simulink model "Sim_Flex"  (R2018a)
settings: Solver=ode3  StartTime=0.0  StopTime=30000  FixedStep=Ts  RelTol=1e-3  EnableMultiTasking=on
InitFcn:
  | run
StopFcn:
  | pl
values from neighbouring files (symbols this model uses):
  atto = [0, 0, -0]'*d2r    [run.m]
  ini = [wb0; atto; Hco]    [run.m]
  Kq1 = I22*ww^2 - 3*wo2*(I11-I33)    [run.m]
  Kq2 = 2*I22*zet*ww    [run.m]
  Kqi = 0.0005    [run.m]
  Kr1 = (0.1*I11*I33*zet^2/Hy0) - sqrt( ((0.01^zet^4*I11^2*I33^2)/Hy0^2)+(4*I11*I33*zet^2) )    [run.m]
  Kr2 = 0.05*Kr1    [run.m]
  Kr3 = 0.04*zet*(Kr2-Hy0) * sqrt(abs(Hy0/(I11*I33)))    [run.m]
  r2d = 180/pi    (= 57.2957795131)    [pl.m]    (also in run.m; plf.m; runf.m; pl2.m)
  Tbs = (wo2)*[-2*I32, 3*I31, -I12]'    [run.m]
  Ts = 0.001    [run.m]    (also in runf.m = 0.0005)
  wb0 = [0.0, -wo, 0.0]'    [run.m]
undefined symbols (not defined in the file or in its folder): Avf, Bvf, Cvf, den, DiscIntNeverNeededParam, Dvf, num, Spacecraft, Wheel_Dynamics
libraries: simulink x3

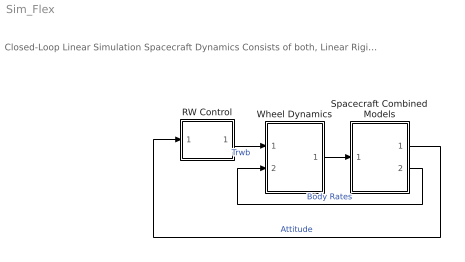
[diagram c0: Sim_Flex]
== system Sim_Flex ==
  note: Closed-Loop Linear Simulation Spacecraft Dynamics Consists of both, Linear Rigid plus Flex Subsystems
  RW Control : Subsystem
  Spacecraft Combined Models : Subsystem
  Wheel Dynamics : Subsystem
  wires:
  RW Control/1(Tc) -> Wheel Dynamics/1(Twi)  "Trwb"
  Wheel Dynamics/1(Tcb) -> Spacecraft Combined Models/1(Trw)
  Spacecraft Combined Models/2(wb) -> Wheel Dynamics/2(wb)  "Body Rates"
  Spacecraft Combined Models/1(attit) -> RW Control/1(atti)  "Attitude"

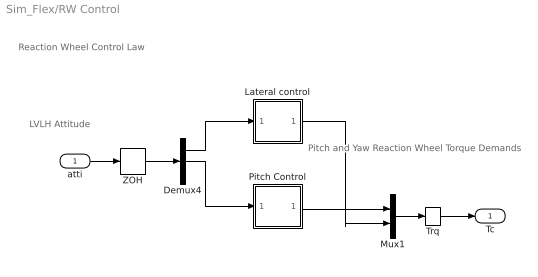
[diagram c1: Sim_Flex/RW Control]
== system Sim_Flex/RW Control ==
  note: Pitch and Yaw Reaction Wheel Torque Demands
  note: LVLH Attitude
  note: Reaction Wheel Control Law
  atti : Inport
  Demux4 : Demux  Outputs=3
  Lateral control : Subsystem
  Mux1 : Mux  Inputs=2
  Pitch Control : Subsystem
  Trq : Memory
  ZOH : ZeroOrderHold  SampleTime=Ts
  Tc : Outport
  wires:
  Demux4/1 -> Lateral control/1(phi)
  Pitch Control/1(Tcy) -> Mux1/1
  Demux4/2 -> Pitch Control/1(the)
  Lateral control/1(Tcz) -> Mux1/2
  atti/1 -> ZOH/1
  Mux1/1 -> Trq/1
  ZOH/1 -> Demux4/1
  Trq/1 -> Tc/1

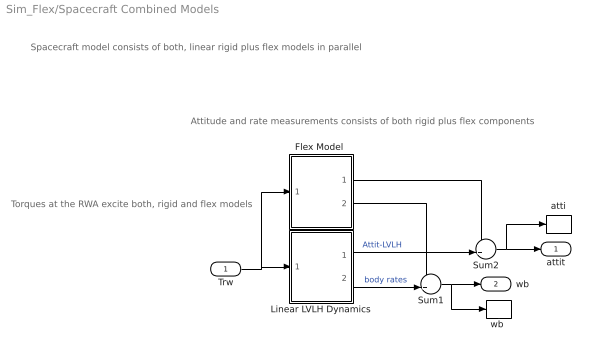
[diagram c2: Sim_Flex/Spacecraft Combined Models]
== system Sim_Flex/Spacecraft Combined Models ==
  note: Torques at the RWA excite both, rigid and flex models
  note: Spacecraft model consists of both, linear rigid plus flex models in parallel
  note: Attitude and rate measurements consists of both rigid plus flex components
  Trw : Inport
  "Flex Model " : Subsystem
  Linear LVLH Dynamics : Subsystem
  Sum1 : Sum  Inputs=++|
  Sum2 : Sum  Inputs=++|
  atti : ToWorkspace  VariableName=atti  SampleTime=-1
  "wb " : ToWorkspace  VariableName=wb  SampleTime=-1
  attit : Outport
  wb : Outport  Port=2
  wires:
  "Flex Model "/2(wb-flx) -> Sum1/1
  Linear LVLH Dynamics/2(wb) -> Sum1/2  "body rates"
  Sum1/1 -> wb/1, "wb "/1
  Sum2/1 -> attit/1, atti/1
  Linear LVLH Dynamics/1(atti-lv) -> Sum2/2  "Attit-LVLH"
  "Flex Model "/1(att-flx) -> Sum2/1
  Trw/1 -> Linear LVLH Dynamics/1(Tsc), "Flex Model "/1(Trwi)

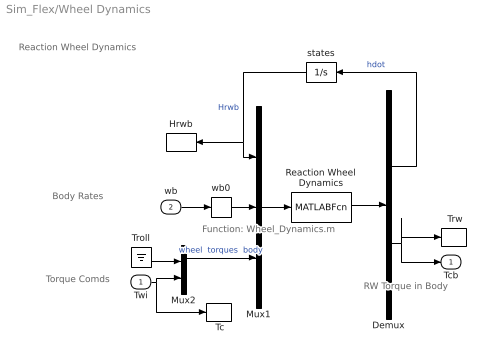
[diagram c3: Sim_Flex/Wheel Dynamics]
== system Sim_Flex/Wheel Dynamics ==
  note: Torque Comds
  note: RW Torque in Body
  note: Body Rates
  note: Reaction Wheel Dynamics
  note: Function: Wheel_Dynamics.m
  Twi : Inport
  wb : Inport  Port=2
  " Tc" : ToWorkspace  VariableName=Tc  SampleTime=-1
  " Trw" : ToWorkspace  VariableName=Trw  SampleTime=-1
  Demux : Demux  Outputs=[3, 3]
  Hrwb : ToWorkspace  VariableName=Hrwb  SampleTime=-1
  Mux1 : Mux  Inputs=[3, 3, 3]
  Mux2 : Mux  Inputs=[1,2]
  Reaction Wheel Dynamics : MATLABFcn  MATLABFcn=Wheel_Dynamics( u(1:3), u(4:6), u(7:9) )  OutputDimensions=3+3
  Troll : Ground
  states : Integrator
  wb0 : Memory  InitialCondition=wb0
  Tcb : Outport
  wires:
  wb0/1 -> Mux1/2
  Troll/1 -> Mux2/1
  Twi/1 -> Mux2/2, " Tc"/1
  Mux1/1 -> Reaction Wheel Dynamics/1
  Reaction Wheel Dynamics/1 -> Demux/1
  Demux/2 -> Tcb/1, " Trw"/1
  Mux2/1 -> Mux1/3  "wheel  torques  body"
  wb/1 -> wb0/1
  Demux/1 -> states/1  "hdot"
  states/1 -> Hrwb/1, Mux1/1  "Hrwb"

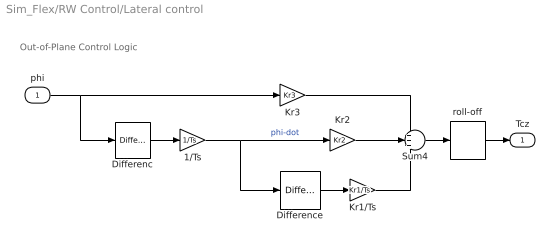
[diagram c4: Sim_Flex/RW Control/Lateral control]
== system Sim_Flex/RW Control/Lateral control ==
  note: Out-of-Plane Control Logic
  phi : Inport
  1/Ts : Gain  Gain=1/Ts
  Differenc : simulink/Discrete/Difference  ICPrevInput=atto(1)  InputProcessing=Inherited  OutMin=[]  OutMax=[]  OutDataType=sfix(16)  OutScaling=2^-10  DoSatur=off
  Difference : simulink/Discrete/Difference  ICPrevInput=0.0  InputProcessing=Inherited  OutMin=[]  OutMax=[]  OutDataType=sfix(16)  OutScaling=2^-10  DoSatur=off
  Kr1/Ts : Gain  Gain=Kr1/Ts
  Kr2 : Gain  Gain=Kr2
  Kr3 : Gain  Gain=Kr3
  Sum4 : Sum  Inputs=+++
  roll-off : DiscreteTransferFcn  Numerator=[num]  Denominator=[den]  SampleTime=Ts
  Tcz : Outport
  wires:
  Kr3/1 -> Sum4/1
  Kr2/1 -> Sum4/2
  Kr1/Ts/1 -> Sum4/3
  phi/1 -> Kr3/1, Differenc/1
  Sum4/1 -> roll-off/1
  Difference/1 -> Kr1/Ts/1
  Differenc/1 -> 1/Ts/1
  1/Ts/1 -> Kr2/1, Difference/1  "phi-dot"
  roll-off/1 -> Tcz/1

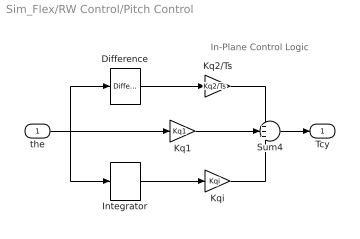
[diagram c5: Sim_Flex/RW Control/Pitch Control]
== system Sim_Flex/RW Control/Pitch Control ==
  note: In-Plane Control Logic
  the : Inport
  Difference : simulink/Discrete/Difference  ICPrevInput=atto(2)  InputProcessing=Inherited  OutMin=[]  OutMax=[]  OutDataType=sfix(16)  OutScaling=2^-10  DoSatur=off
  Integrator : DiscreteIntegrator  InitialCondition=atto(2)  SampleTime=Ts  ICPrevOutput=DiscIntNeverNeededParam  ICPrevScaledInput=DiscIntNeverNeededParam
  Kq1 : Gain  Gain=Kq1
  Kq2/Ts : Gain  Gain=Kq2/Ts
  Kqi : Gain  Gain=Kqi
  Sum4 : Sum  Inputs=+++
  Tcy : Outport
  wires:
  Kq1/1 -> Sum4/2
  Sum4/1 -> Tcy/1
  Kq2/Ts/1 -> Sum4/1
  the/1 -> Kq1/1, Integrator/1, Difference/1
  Kqi/1 -> Sum4/3
  Integrator/1 -> Kqi/1
  Difference/1 -> Kq2/Ts/1

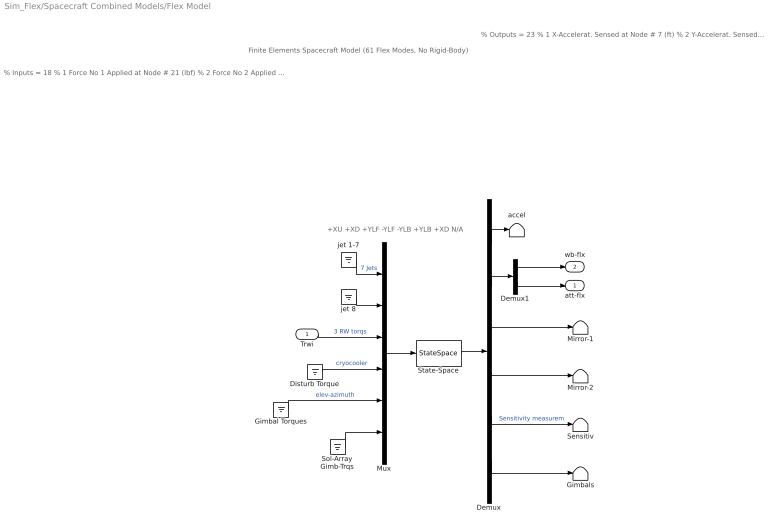
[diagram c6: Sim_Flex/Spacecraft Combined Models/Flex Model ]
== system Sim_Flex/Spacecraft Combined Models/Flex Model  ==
  note: +XU +XD +YLF -YLF -YLB +YLB +XD N/A
  note: % Outputs = 23 % 1 X-Accelerat. Sensed at Node # 7 (ft) % 2 Y-Accelerat. Sensed at Node # 7 (ft) % 3 X-Rot. Rate Sensed at Node # 6 (radian) % 4 Y-Rot. Rate Sensed at Node # 6 (radian) % 5 Z-Rot. Rate Sensed at Node # 6 (radian) % 6 X-Rotation Sensed at Node # 6 (radian) % 7 Y-Rotation Sensed at Node # 6 (radian) % 8 Z-Rotation Sensed at Node # 6 (radian) % 9 Y-Rotation Sensed at Node # 9 (radian) % 10 Z-Rotation Sensed at Node # 9 (radian) % 11 Y-Rotation Sensed at Node # 10 (radian) % 12 Z-Rotation Sensed at Node # 10 (radian) % 13 X-Rotation Sensed at Node # 11 (radian) % 14 Y-Rotation Sensed at Node # 12 (radian) % 15 Z-Rotation Sensed at Node # 13 (radian) % 16 Rotation Angle at Gimbal No 1 in (radians) % 17 Rotation Rate at Gimbal No 1 in (rad/sec) % 18 Rotation Angle at Gimbal No 2 in (radians) % 19 Rotation Rate at Gimbal No 2 in (rad/sec) % 20 Rotation Angle at Gimbal No 3 in (radians) % 21 Rotation Rate at Gimbal No 3 in (rad/sec) % 22 Rotation Angle at Gimbal No 4 in (radians) % 23 Rotation Rate at Gimbal No 4 in (rad/sec)
  note: % Inputs = 18 % 1 Force No 1 Applied at Node # 21 (lbf) % 2 Force No 2 Applied at Node # 22 (lbf) % 3 Force No 3 Applied at Node # 23 (lbf) % 4 Force No 4 Applied at Node # 24 (lbf) % 5 Force No 5 Applied at Node # 25 (lbf) % 6 Force No 6 Applied at Node # 26 (lbf) % 7 Force No 7 Applied at Node # 27 (lbf) % 8 Force No 8 Applied at Node # 28 (lbf) % 9 Torque No 1 Applied at Node # 17 (ft-lb) % 10 Torque No 2 Applied at Node # 18 (ft-lb) % 11 Torque No 3 Applied at Node # 19 (ft-lb) % 12 Torque No 4 Applied at Node # 8 (ft-lb) % 13 Torque No 5 Applied at Node # 8 (ft-lb) % 14 Torque No 6 Applied at Node # 8 (ft-lb) % 15 Control Torque at Gimbal No 1 in (ft-lb) % 16 Control Torque at Gimbal No 2 in (ft-lb) % 17 Control Torque at Gimbal No 3 in (ft-lb) % 18 Control Torque at Gimbal No 4 in (ft-lb)
  note: Finite Elements Spacecraft Model (61 Flex Modes, No Rigid-Body)
  Trwi : Inport
  Demux : Demux  Outputs="[2, 6, 2,2,3,  8]"
  Demux1 : Demux  Outputs=[3, 3]
  Disturb Torque : Ground
  Gimbal Torques : Ground
  Gimbals : Terminator
  Mirror-1 : Terminator
  Mirror-2 : Terminator
  Mux : Mux  Inputs=[7,1,3,3,2,2]
  Sensitiv : Terminator
  Sol-Array Gimb-Trqs : Ground
  State-Space : StateSpace  A=Avf  B=Bvf  C=Cvf  D=Dvf  InitialCondition=0
  accel : Terminator
  jet 1-7 : Ground
  jet 8 : Ground
  att-flx : Outport
  wb-flx : Outport  Port=2
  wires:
  Demux1/2 -> att-flx/1
  Demux/4 -> Mirror-2/1
  Demux/3 -> Mirror-1/1
  Demux/5 -> Sensitiv/1  "Sensitivity measurem"
  Sol-Array Gimb-Trqs/1 -> Mux/6
  Disturb Torque/1 -> Mux/4  "cryocooler"
  Trwi/1 -> Mux/3  "3 RW torqs"
  jet 8/1 -> Mux/2
  jet 1-7/1 -> Mux/1  "7 Jets"
  Mux/1 -> State-Space/1
  Demux1/1 -> wb-flx/1
  Demux/2 -> Demux1/1
  State-Space/1 -> Demux/1
  Demux/1 -> accel/1
  Gimbal Torques/1 -> Mux/5  "elev-azimuth"
  Demux/6 -> Gimbals/1

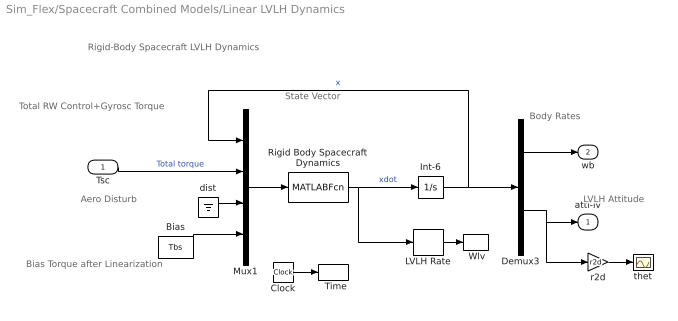
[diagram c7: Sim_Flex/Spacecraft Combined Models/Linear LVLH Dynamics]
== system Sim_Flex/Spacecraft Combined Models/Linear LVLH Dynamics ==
  note: LVLH Attitude
  note: Body Rates
  note: Bias Torque after Linearization
  note: Aero Disturb
  note: Total RW Control+Gyrosc Torque
  note: Rigid-Body Spacecraft LVLH Dynamics
  note: State Vector
  Tsc : Inport
  "  Time" : ToWorkspace  VariableName=time  SampleTime=-1
  "  Wlv " : ToWorkspace  VariableName=Wlv  SampleTime=-1
  Bias : Constant  Value=Tbs
  Clock : Clock
  Demux3 : Demux  Outputs=[3, 3]
  Int-6 : Integrator  InitialCondition=ini
  LVLH Rate : Selector  InputPortWidth=6  IndexOptions=Index vector (dialog)  Indices=[4:6]  OutputSizes=1
  Mux1 : Mux  Inputs=[6, 3, 3, 3]
  Rigid Body Spacecraft Dynamics : MATLABFcn  MATLABFcn=Spacecraft( u(1:6), u(7:9) , u(10:12), u(13:15) )  OutputDimensions=6
  dist : Ground
  r2d : Gain  Gain=r2d
  thet : Scope
  atti-lv : Outport
  wb : Outport  Port=2
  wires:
  dist/1 -> Mux1/3
  Bias/1 -> Mux1/4
  LVLH Rate/1 -> "  Wlv "/1
  Rigid Body Spacecraft Dynamics/1 -> LVLH Rate/1, Int-6/1  "xdot"
  Tsc/1 -> Mux1/2  "Total torque"
  r2d/1 -> thet/1
  Int-6/1 -> Demux3/1, Mux1/1  "x"
  Demux3/1 -> wb/1
  Demux3/2 -> atti-lv/1, r2d/1
  Mux1/1 -> Rigid Body Spacecraft Dynamics/1
  Clock/1 -> "  Time"/1
